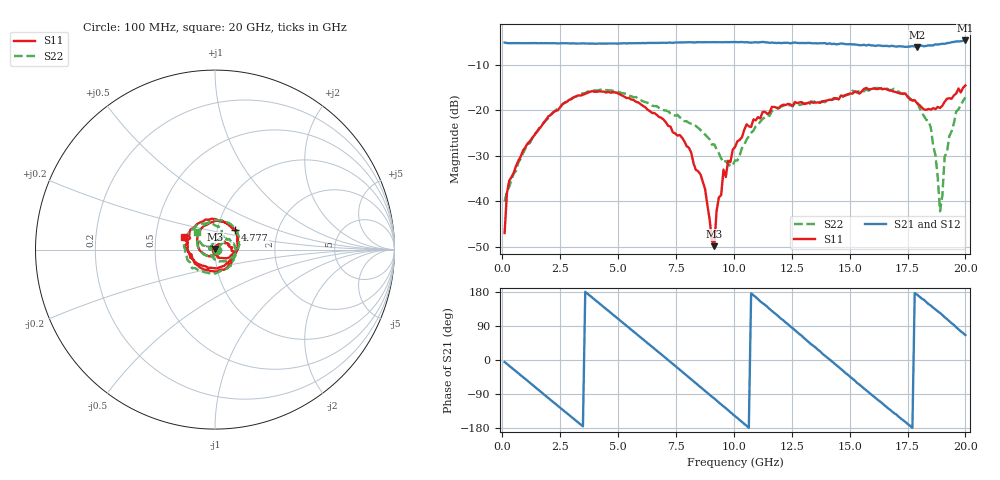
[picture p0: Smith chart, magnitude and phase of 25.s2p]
!Agilent Technologies,N5230C,MY49001569,A.09.33.09
!Agilent N5230C: A.09.33.09
!Date: Monday, July 27, 2015 17:15:30
!Correction: S11(Full 2 Port(1,2))
!S21(Full 2 Port(1,2))
!S12(Full 2 Port(1,2))
!S22(Full 2 Port(1,2))
!S2P File: Measurements: S11, S21, S12, S22:
# Hz S  dB  R 50
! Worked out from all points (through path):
!   201 points, 100 MHz to 20 GHz, reference 50 ohm
!   highest |S21| = -4.63 dB at 20 GHz (marker M1); lowest = -6.0 dB at 17.91 GHz (marker M2)
!   group delay of S21, straight-line fit = 141 ps
!   lowest |S11| = -49.9 dB at 9.155 GHz (marker M3), VSWR 1.01, Z = 50 + j0.32 ohm
!   |S11| at or under -10 dB: start of sweep to end of sweep
!   |S22| runs from -42.2 to -15.1 dB; largest |S21 - S12| = 0.03
!   S11 on the Smith chart (normalised r, x): 100 MHz: 1.01, -0.00; 4.777 GHz: 1.22, +0.28; 20 GHz: 0.70, +0.10
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1e8  -46.99 -18.6  -5.11 -5.3  -5.20 -5.2  -40.06 -6.0
2.99e8  -35.51 -38.7  -5.23 -15.3  -5.22 -15.1  -36.84 -37.1
8.96e8  -28.81 -102.9  -5.22 -45.1  -5.23 -45.4  -29.42 -106.7
2.09e9  -21.03 177.7  -5.25 -105.2  -5.26 -105.6  -20.98 177.6
3.483e9  -16.57 103.8  -5.26 -175.1  -5.32 -175.6  -16.27 107.3
4.7765e9  -16.04 44.1  -5.30 120.2  -5.34 120.0  -15.70 51.0
6.7665e9  -21.43 -33.0  -5.17 20.0  -5.14 19.5  -19.45 -21.8
8.1595e9  -29.31 -70.5  -5.02 -51.0  -5.04 -51.6  -22.96 -65.3
8.7565e9  -37.29 -106.8  -5.00 -81.3  -5.08 -82.2  -25.34 -94.8
9.1545e9  -49.89 91.8  -5.00 -101.4  -5.07 -102.8  -27.49 -115.7
9.5525e9  -33.05 77.0  -5.04 -122.2  -5.07 -122.9  -31.50 -151.0
1.005e10  -28.06 53.0  -4.97 -148.2  -5.01 -148.8  -31.01 140.7
1.09455e10  -22.20 18.0  -5.03 165.9  -4.92 164.6  -23.53 62.0
1.19405e10  -19.52 -18.7  -5.14 114.4  -5.15 113.0  -19.51 17.6
1.3433e10  -18.31 -93.2  -5.26 37.2  -5.27 36.4  -18.21 -50.3
1.53235e10  -15.89 160.6  -5.58 -60.5  -5.61 -60.6  -16.13 -152.6
1.67165e10  -15.64 84.5  -5.93 -129.8  -5.82 -130.6  -15.56 137.5
1.79105e10  -18.44 -6.7  -6.05 172.7  -5.94 170.5  -18.16 72.2
1.85075e10  -19.87 -71.1  -5.73 143.6  -5.80 141.7  -23.82 40.3
1.89055e10  -19.49 -118.7  -5.45 124.1  -5.52 121.8  -42.21 55.1
1.91045e10  -18.13 -140.3  -5.37 112.9  -5.36 112.1  -30.18 179.0
2e10  -14.54 158.5  -4.63 65.7  -4.64 63.8  -17.15 135.4
